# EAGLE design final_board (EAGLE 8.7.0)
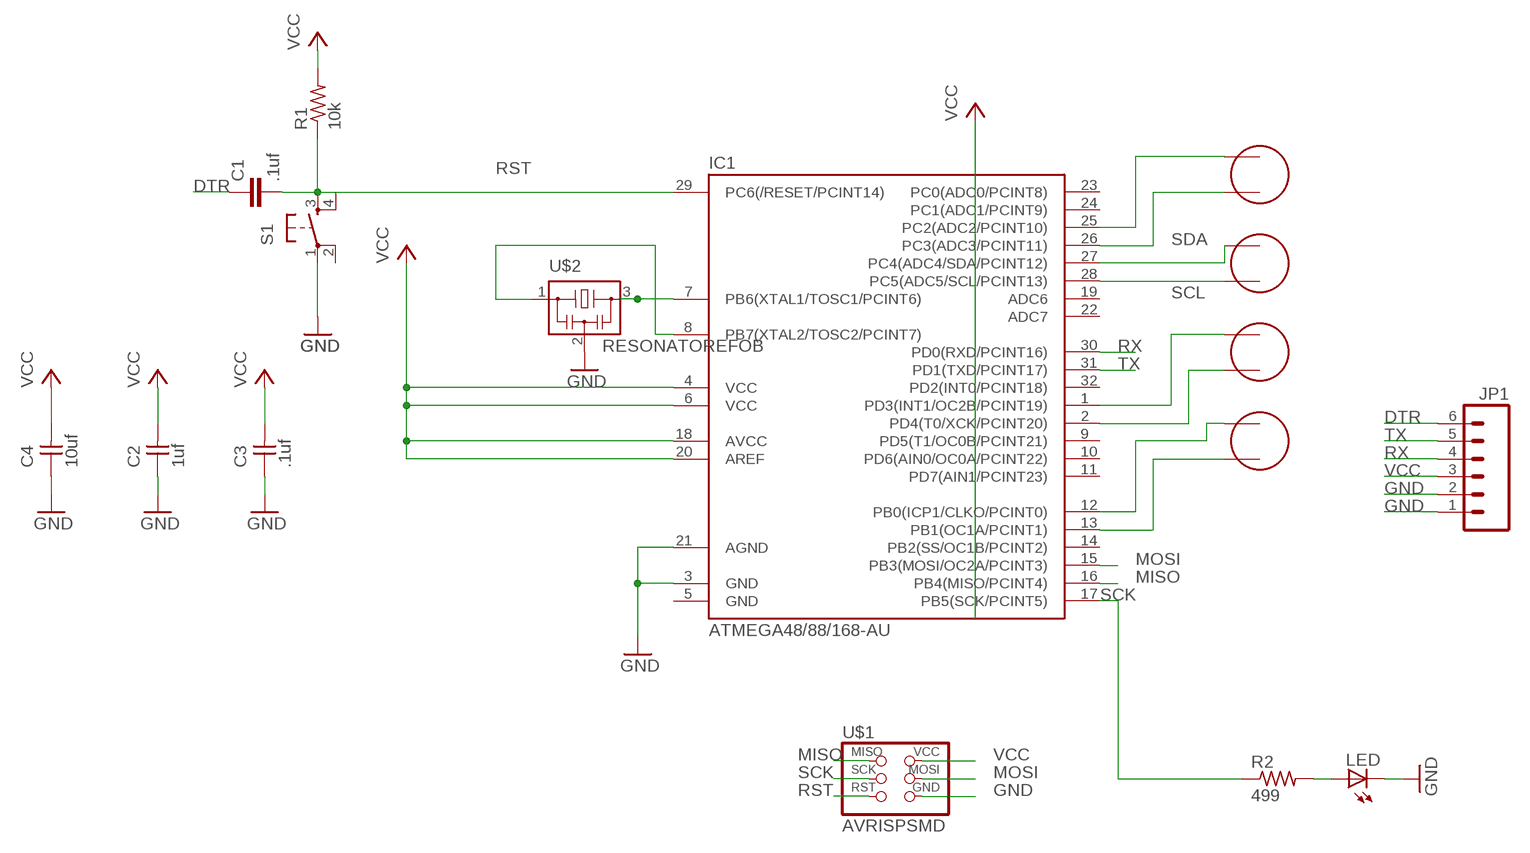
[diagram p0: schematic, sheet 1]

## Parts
C1  .1uf  C-EUC1206  [C1206]
C2  1uf  UNPOLARIZED_CAPACITOR1206  [1206]
C3  .1uf  UNPOLARIZED_CAPACITOR1206  [1206]
C4  10uf  UNPOLARIZED_CAPACITOR1206  [1206]
IC1  ATMEGA48/88/168-AU  [TQFP32-08]
JP1  M06SMD  [1X06-SMD]
LED  LED1206  [1206]
R1  10k  RESISTOR1206  [1206]
R2  499  RESISTOR1206  [1206]
S1  6MM_SWITCH6MM_SWITCH  [6MM_SWITCH]
U$1  AVRISPSMD  [2X03SMD]
U$2  RESONATOREFOB  [EFOBM]
U$3  ELECTRET  [ELECTRET_2742PBJ-A]
U$4  ELECTRET  [ELECTRET_2742PBJ-A]
U$5  ELECTRET  [ELECTRET_2742PBJ-A]
U$6  ELECTRET  [ELECTRET_2742PBJ-A]

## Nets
DTR: C1.1 JP1.6
GND: C2.1 C3.1 C4.1 IC1.3(GND) IC1.21(AGND) JP1.1 JP1.2 LED.2(C) S1.1(P) U$1.6(GND) U$2.2
MISO: IC1.16(PB4(MISO/PCINT4)) U$1.1(MISO)
MOSI: IC1.15(PB3(MOSI/OC2A/PCINT3)) U$1.4(MOSI)
N$1: IC1.8(PB7(XTAL2/TOSC2/PCINT7)) U$2.1
N$2: IC1.1(PD3(INT1/OC2B/PCINT19)) U$4.P$1
N$3: IC1.2(PD4(T0/XCK/PCINT20)) U$4.P$2
N$4: IC1.12(PB0(ICP1/CLKO/PCINT0)) U$5.P$1
N$5: IC1.13(PB1(OC1A/PCINT1)) U$5.P$2
N$6: IC1.26(PC3(ADC3/PCINT11)) U$6.P$2
N$7: IC1.25(PC2(ADC2/PCINT10)) U$6.P$1
N$9: IC1.7(PB6(XTAL1/TOSC1/PCINT6)) U$2.3
N$23: LED.1(A) R2.2
RST: C1.2 IC1.29(PC6(/RESET/PCINT14)) R1.1 S1.3(S) U$1.5(RST)
RX: IC1.30(PD0(RXD/PCINT16)) JP1.4
SCK: IC1.17(PB5(SCK/PCINT5)) R2.1 U$1.3(SCK)
SCL: IC1.28(PC5(ADC5/SCL/PCINT13)) U$3.P$2
SDA: IC1.27(PC4(ADC4/SDA/PCINT12)) U$3.P$1
TX: IC1.31(PD1(TXD/PCINT17)) JP1.5
VCC: C2.2 C3.2 C4.2 IC1.4(VCC) IC1.6(VCC) IC1.18(AVCC) IC1.20(AREF) JP1.3 R1.2 U$1.2(VCC)
Unconnected: IC1.9(PD5(T1/OC0B/PCINT21)) IC1.10(PD6(AIN0/OC0A/PCINT22)) IC1.11(PD7(AIN1/PCINT23)) IC1.14(PB2(SS/OC1B/PCINT2)) IC1.19(ADC6) IC1.22(ADC7) IC1.23(PC0(ADC0/PCINT8)) IC1.24(PC1(ADC1/PCINT9)) IC1.32(PD2(INT0/PCINT18)) S1.2(P1) S1.4(S1)

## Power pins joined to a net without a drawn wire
GND: IC1.5(GND)

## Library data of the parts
C1 = rcl:C-EU: CAPACITOR, European symbol
C2-C4 = ng:UNPOLARIZED_CAPACITOR: unpolarized_capacitor
IC1 = atmega8:ATMEGA48/88/168
JP1 = SparkFun:M06: Header 6 Standard 6-pin 0.1" header. Use with straight break away headers (SKU : PRT-00116), right angle break away headers (PRT-00553), swiss pins (PRT-00743), machine pins (PRT-00117), and female headers (PRT-00115). Molex polarized connector foot print use with SKU : PRT-08094 with associated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
LED = ng:LED
R1 R2 = ng:RESISTOR
S1 = ng:6MM_SWITCH: OMRON SWITCH
U$1 = fab:AVRISP
U$2 = fab:RESONATOR
U$3-U$6 = fab:ELECTRET

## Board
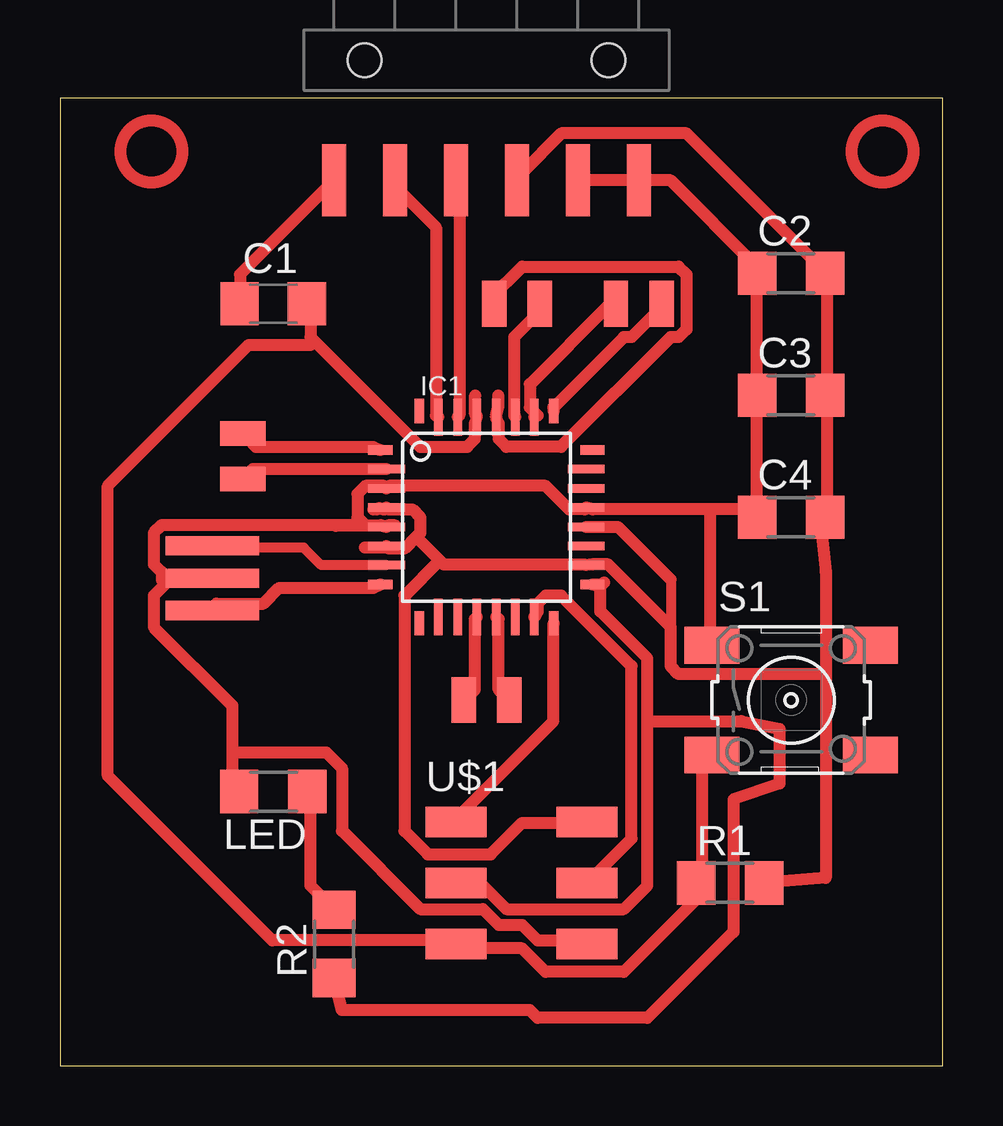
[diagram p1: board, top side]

Size 36.81 x 40.31 mm. Coordinates in mm from the lower left corner, seen from the top.
Outline: 0,0 36.81,0 36.81,40.31 0,40.31 0,0
Copper layers (1*16): Top 0.035mm / dielectric 1.5mm / Bottom 0.035mm
Design rules "default *": minimum track width 0.5mm, minimum drill 0.5mm, track to track 0.153mm, track to pad 0.153mm, pad to pad 0.153mm, via to via 0.153mm, smd to smd 0.153mm, copper to edge 40mil, drill to drill 6mil, minimum pad ring 10mil, minimum via ring 8mil, stop-mask expansion 4mil, vias tented up to drill 0mil, thermal gap 10mil

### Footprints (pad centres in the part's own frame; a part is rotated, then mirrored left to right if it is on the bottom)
C1206 = smd 1.6 x 1.8: 1 -1.4,0; 2 1.4,0
1206 = smd 1.6 x 1.803: 1 -1.422,0; 2 1.422,0
TQFP32-08 = smd 1.016 x 0.406: 1 -4.42,2.8; 8 -4.42,-2.8; 17 4.42,-2.8; 24 4.42,2.8 | smd 1.524 x 0.356: 2 -4.166,2; 3 -4.166,1.2; 4 -4.166,0.4; 5 -4.166,-0.4; 6 -4.166,-1.2; 7 -4.166,-2; 18 4.166,-2; 19 4.166,-1.2; 20 4.166,-0.4; 21 4.166,0.4; 22 4.166,1.2; 23 4.166,2 | smd 0.406 x 1.016: 9 -2.8,-4.42; 16 2.8,-4.42; 25 2.8,4.42; 32 -2.8,4.42 | smd 0.356 x 1.524: 10 -2,-4.166; 11 -1.2,-4.166; 12 -0.4,-4.166; 13 0.4,-4.166; 14 1.2,-4.166; 15 2,-4.166; 26 2,4.166; 27 1.2,4.166; 28 0.4,4.166; 29 -0.4,4.166; 30 -1.2,4.166; 31 -2,4.166
1X06-SMD = smd 1 x 3: 1 -6.35,5; 2 -3.81,5; 3 -1.27,5; 4 1.27,5; 5 3.81,5; 6 6.35,5 | hole 1.4: -5.08,0; 5.08,0
6MM_SWITCH = smd 2.286 x 1.524: 1 -3.302,2.286; 2 3.302,2.286; 3 -3.302,-2.286; 4 3.302,-2.286
2X03SMD = smd 2.54 x 1.27: 1 -2.54,2.54; 2 2.92,2.54; 3 -2.54,0; 4 2.92,0; 5 -2.54,-2.54; 6 2.92,-2.54
EFOBM = smd 0.8 x 3.9: 1 -1.35,0; 2 0,0; 3 1.35,0
ELECTRET_2742PBJ-A = smd 1.016 x 1.905: P$1 -0.953,0; P$2 0.953,0

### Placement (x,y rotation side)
C1  8.89,31.75 0 top
C2  30.48,33.02 0 top
C3  30.48,27.94 0 top
C4  30.48,22.86 0 top
IC1  17.78,22.86 0 top
JP1  17.78,41.91 180 top
LED  8.89,11.43 180 top
R1  27.94,7.62 0 top
R2  11.43,5.08 90 top
S1  30.48,15.24 0 top
U$1  19.05,7.62 0 top
U$2  6.35,20.32 90 top
U$3  19.05,31.75 180 top
U$4  7.62,25.4 270 top
U$5  17.78,15.24 0 top
U$6  24.13,31.75 180 top

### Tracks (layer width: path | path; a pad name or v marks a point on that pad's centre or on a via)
DTR
  Top 0.5: C1.1 7.51,32 7.51,32.98 11.42,36.89 JP1.6
GND
  Top 0.406: IC1.5 11.5,22.46 11.43,22.53
  Top 0.5: 7.18,13.06 7.18,15.02 3.92,18.28 3.92,19.59 4.4,20.08 | 7.18,13.06 7.18,11.75 LED.2 | 4.4,20.08 4.57,20.24 6.2,20.24 U$2.2 | 7.18,13.06 11.1,13.06 11.75,12.41 11.75,9.79 15.02,6.53 17.63,6.53 18.28,5.88 19.26,5.88 19.91,5.22 21.87,5.22 U$1.6 | JP1.2 21.87,36.89 23.83,36.89 JP1.1 24.16,36.89 25.46,36.89 29.06,33.3 C2.1 29.06,32.98 29.06,28.08 C3.1 29.06,27.75 29.06,23.18 | 12.57,22.69 12.4,22.86 12.4,23.83 12.73,24.16 | 12.57,22.69 12.73,22.53 13.38,22.53 IC1.5 | 29.06,23.18 27.1,23.18 | 27.1,23.18 22.2,23.18 IC1.21 21.87,23.18 21.22,23.18 20.24,24.16 13.71,24.16 IC1.3 | 29.06,23.18 C4.1 | 27.1,23.18 27.1,17.63 S1.1 | 4.4,20.08 4.24,20.24 4.24,20.57 3.92,20.9 3.92,22.2 4.24,22.53 11.43,22.53 12.4,22.53 12.57,22.69
  Top 0.508: IC1.3 13.51,24.16 12.73,24.16 | 13.97,22.52 13.74,22.52 13.67,22.52 IC1.5
MISO
  Top 0.5: IC1.16 20.57,18.28 20.57,14.37 16.65,10.45 U$1.1
MOSI
  Top 0.5: IC1.15 19.91,18.94 19.91,19.26 20.24,19.59 20.89,19.59 23.83,16.65 23.83,9.47 22.2,7.84 U$1.4
N$1
  Top 0.5: IC1.8 13.06,19.92 9.14,19.92 8.49,19.26 6.53,19.26 U$2.1
N$2
  Top 0.5: IC1.1 13.06,25.79 8.16,25.79 7.83,26.12 U$4.P$1
N$3
  Top 0.406: 8.03,24.86 U$4.P$2
  Top 0.508: IC1.2 8.03,24.86
N$4
  Top 0.5: IC1.12 17.3,18.61 17.3,15.67 16.98,15.34 U$5.P$1
N$5
  Top 0.5: IC1.13 18.28,18.61 18.28,15.67 18.61,15.34 U$5.P$2
N$6
  Top 0.5: IC1.26 19.91,27.1 19.59,27.43 19.59,28.41 22.85,31.67 U$6.P$2
N$7
  Top 0.5: IC1.25 20.57,27.43 23.5,30.36 23.83,30.36 25.14,31.67 U$6.P$1
N$9
  Top 0.406: U$2.3 6.43,21.59 10.16,21.59 10.89,20.86 IC1.7
N$23
  Top 0.5: LED.1 10.45,11.43 10.45,7.51 11.42,6.53 R2.2
RST
  Top 0.5: 10.61,30.2 10.45,30.36 10.45,31.67 C1.2 | 10.61,30.2 15.02,25.79 16.98,25.79 17.3,26.12 17.3,26.77 IC1.29 | S1.3 27.1,12.73 26.77,12.41 26.77,7.84 R1.1 26.44,7.51 26.44,6.86 23.5,3.92 20.24,3.92 19.26,4.9 16.65,4.9 U$1.5 16.32,5.22 8.85,5.22 1.99,12.08 1.99,24.16 7.87,30.04 10.45,30.04 10.61,30.2
  Top 0.508: IC1.29 17.38,27.07 17.31,27.14 17.31,27.94
RX
  Top 0.5: IC1.30 16.65,27.1 16.65,36.89 JP1.4
SCK
  Top 0.5: 24.48,14.37 24.48,7.51 23.5,6.53 18.61,6.53 17.63,7.51 16.65,7.51 U$1.3 | 24.48,14.37 24.48,16.98 22.53,18.94 22.53,19.92 IC1.17 | 24.48,14.37 28.4,14.37 30,14.04 30,11.75 28.08,11.1 28.08,5.59 24.48,2 19.91,2 19.59,2.32 11.75,2.32 R2.1
  Top 0.508: IC1.17 22.6,20.06 22.68,20.14
SCL
  Top 0.5: IC1.28 18.28,26.77 18.28,26.12 18.61,25.79 20.89,25.79 25.46,30.36 25.79,30.36 26.12,30.69 26.12,32.98 25.79,33.3 19.26,33.3 17.95,32 U$3.P$2
  Top 0.508: IC1.28 18.18,27.07 18.28,27.48 18.28,27.94
SDA
  Top 0.5: IC1.27 18.93,27.1 18.93,30.36 20.24,31.67 U$3.P$1
TX
  Top 0.5: IC1.31 15.67,27.1 15.67,34.94 13.71,36.89 JP1.5
VCC
  Top 0.406: 25.46,20.25 25.46,17.78
  Top 0.5: 14.85,22.04 15.02,22.2 15.02,22.86 14.69,23.18 13.71,23.18 IC1.4 | 14.85,22.04 14.36,21.55 13.71,21.55 IC1.6 | 14.85,22.04 15.83,21.06 | 15.83,21.06 16,20.9 21.87,20.9 IC1.18 22.2,20.9 22.85,20.9 25.46,18.28 25.46,17.78 25.46,16.65 25.79,16.32 31.92,16.32 | 15.83,21.06 14.36,19.59 14.36,9.79 15.34,8.81 17.95,8.81 19.26,10.12 21.87,10.12 U$1.2 | 31.92,16.32 31.92,20.57 31.67,22.86 C4.2 31.99,23.18 31.99,27.75 C3.2 31.99,28.08 31.99,32.98 C2.2 31.67,33.3 26.12,38.85 20.89,38.85 19.26,37.22 JP1.3 | 31.92,16.32 31.92,7.84 R1.2
  Top 0.508: IC1.20 23.26,22.46 25.46,20.25 | IC1.6 13.54,21.59 12.7,21.59 | IC1.4 13.54,23.19 13.48,23.19 13.31,23.24 13.22,23.19 13.06,23.19
(copper drawn outside any net)
  shapes: Top circle x2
